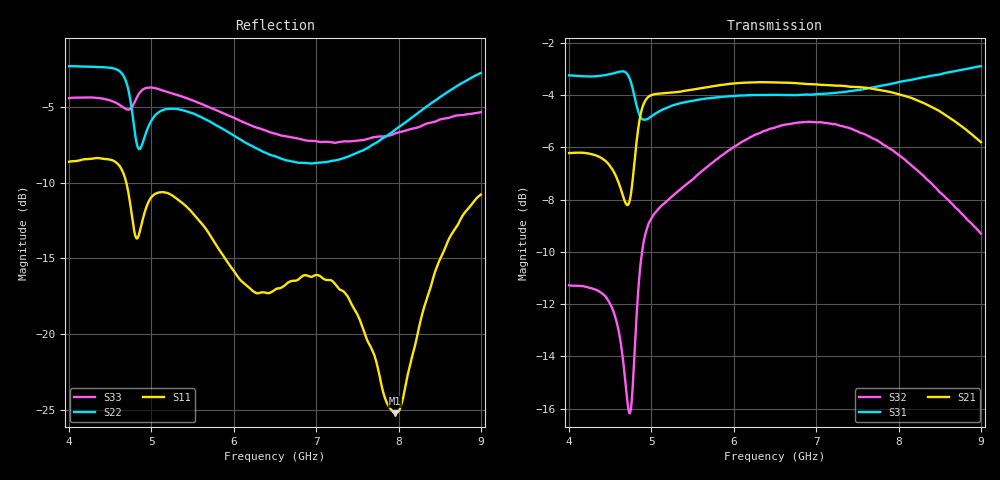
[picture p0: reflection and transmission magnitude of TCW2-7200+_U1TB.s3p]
!Created: 08-09-2021 at 09:48:20
!MODEL: TCW2-7200+
!S/N: U1TB
# MHZ S DB R 50
!Frequency
!  S11 dB  S11 DEG  S12 dB  S12 DEG  S13 dB  S13 DEG
!  S21 dB  S21 DEG  S22 dB  S22 DEG  S23 dB  S23 DEG
!  S31 dB  S31 DEG  S32 dB  S32 DEG  S33 dB  S33 DEG
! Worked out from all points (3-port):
!   501 points, 4 GHz to 9 GHz, reference 50 ohm
!   strongest paths, dB at 4 GHz, 5.25 GHz, 6.5 GHz, 7.75 GHz, 9 GHz:
!     S21: -6.2, -3.9, -3.5, -3.8, -5.8
!     S31: -3.2, -4.4, -4.0, -3.7, -2.9
!     S32: -11.3, -7.9, -5.2, -5.8, -9.3
!   lowest |S11| = -25.3 dB at 7.96 GHz (marker M1), VSWR 1.12, Z = 45.8 + j3.06 ohm
!   |S11| at or under -10 dB: 4.694 GHz to end of sweep
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4000  -8.62 68.2  -6.28 127.5  -3.30 -48.5
      -6.22 127.5  -2.31 9.7  -11.28 22.8
      -3.25 -48.5  -11.28 22.8  -4.42 16.1
4560  -8.63 32.0  -7.11 105.0  -3.21 -73.0
      -7.05 105.0  -2.49 -8.1  -12.49 13.9
      -3.15 -73.1  -12.49 13.8  -4.71 7.9
4740  -11.34 16.5  -8.04 116.2  -3.47 -86.4
      -7.98 116.2  -4.44 -24.2  -16.18 36.6
      -3.41 -86.5  -16.18 36.6  -5.13 11.6
4840  -13.57 35.9  -5.32 118.5  -4.70 -90.1
      -5.26 118.5  -7.74 -12.8  -11.45 56.2
      -4.63 -90.2  -11.45 56.2  -4.19 13.3
4990  -11.03 41.2  -4.08 102.6  -4.90 -88.1
      -4.01 102.6  -5.99 3.8  -8.77 40.5
      -4.83 -88.2  -8.77 40.4  -3.71 6.9
6500  -17.08 69.9  -3.58 39.8  -4.06 -142.3
      -3.52 39.8  -8.26 -11.4  -5.24 -6.2
      -3.99 -142.3  -5.24 -6.2  -6.76 -14.4
7340  -17.24 85.5  -3.72 11.0  -3.95 -172.7
      -3.65 11.0  -8.36 -28.9  -5.21 -34.4
      -3.88 -172.8  -5.21 -34.5  -7.27 -35.6
7960  -25.25 142.4  -3.99 -11.6  -3.60 165.2
      -3.93 -11.6  -6.50 -57.9  -6.19 -55.3
      -3.54 165.1  -6.19 -55.4  -6.75 -61.8
8470  -15.52 -167.4  -4.63 -31.7  -3.29 146.6
      -4.57 -31.7  -4.48 -81.7  -7.61 -70.8
      -3.23 146.5  -7.61 -70.8  -5.91 -82.9
9000  -10.79 -179.7  -5.86 -52.7  -2.96 127.4
      -5.80 -52.7  -2.75 -101.2  -9.30 -84.1
      -2.89 127.4  -9.30 -84.2  -5.35 -100.4
